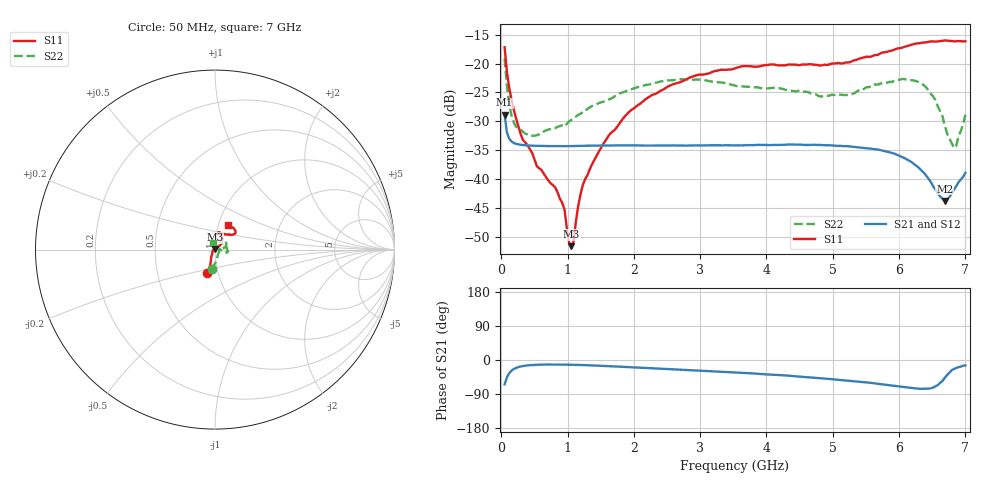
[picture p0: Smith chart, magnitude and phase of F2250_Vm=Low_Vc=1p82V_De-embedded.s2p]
! Integrated Device Technology
! Corporate Headquarters
! 6024 Silver Creek Valley Road
! San Jose, CA 95138  USA
! Phone:  1-408-284-8200
! Toll Free:  1-800-223-1366
! Webpage:  http://www.idt.com/
! Timing and RF Division
! 515 Groton Road, Suite 102
! Westford, MA 01886-6024
! Device:  F2250
! Description: Voltage Variable RF Attenuator
! Frequency:  50.0 -  6000.00 MHz
! Package:  3x3 mm Thin QFN Plastic Package: 16 pin
! Ports:  2 RF, 3 DC
!  Pin  1  = GND
!  Pin  2  = NC
!  Pin  3  = RF1  = Port 1
!  Pin  4  = NC
!  Pin  5  = GND
!  Pin  6  = GND
!  Pin  7  = GND
!  Pin  8  = GND
!  Pin  9  = NC
!  Pin 10  = RF2  = Port 2
!  Pin 11  = NC
!  Pin 12  = GND
!  Pin 13  = GND
!  Pin 14  = VCNTRL
!  Pin 15  = VDD
!  Pin 16  = VMODE
! Vcntrl:  1.820 Volts
! Vmode:  +0.000 Volts
! Vdd:  +3.30  Volts
! Current:  1.186 mA
! Data:  The device was measured on a the F2250 evaluation board which has
!  individual transmission lines to the RF pins.  Data was collected
!  using a calibrated network analyzer.  The evaluation board was
!  de-embedded using a TRL calibration technique.
!  The reference plane is the edge of the package pin.
! Misc:  SN 10
!  Action Tracker AT0258
! Date Measured:  2014-11-26
! Date:  2015-10-15  MJV
! Note:
!  Integrated Device Technology supplies this data as a sample of measured
!  data at the package pin for this product.  Your particular data for this
!  product may vary.
!  Data was taken at 25 degrees C.
!  Integrated Device Technology reserves the right to change this data at anytime.
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# GHz S dB R 50
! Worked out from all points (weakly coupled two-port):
!   201 points, 50 MHz to 7 GHz, reference 50 ohm
!   highest |S21| = -28.84 dB at 50 MHz (marker M1); lowest = -43.8 dB at 6.687 GHz (marker M2)
!   lowest |S11| = -51.6 dB at 1.058 GHz (marker M3), VSWR 1.01, Z = 49.9 + j0.233 ohm
!   |S11| at or under -10 dB: start of sweep to end of sweep
!   |S22| runs from -34.6 to -19.1 dB; largest |S21 - S12| = 5.5e-05
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0.05  -17.17 -108.4  -28.84 -64.2  -28.84 -64.2  -19.11 -100.0
0.1195  -24.20 -111.4  -33.00 -34.7  -33.01 -34.7  -26.93 -73.8
0.22375  -29.54 -121.5  -33.90 -20.8  -33.90 -20.8  -30.94 -50.6
0.5365  -37.77 -154.4  -34.25 -12.6  -34.24 -12.6  -32.40 -9.2
0.91875  -44.10 158.0  -34.30 -12.2  -34.29 -12.2  -30.70 -0.4
0.9535  -45.28 170.4  -34.30 -12.2  -34.29 -12.2  -30.90 1.8
1.023  -51.05 141.9  -34.29 -12.4  -34.29 -12.4  -30.02 4.1
1.05775  -51.61 117.1  -34.28 -12.5  -34.28 -12.5  -29.75 5.0
1.0925  -50.74 83.0  -34.27 -12.7  -34.27 -12.7  -29.50 4.7
1.162  -44.50 53.3  -34.26 -13.0  -34.26 -13.0  -28.88 4.0
1.2315  -40.95 42.1  -34.24 -13.3  -34.25 -13.3  -28.39 4.0
1.6485  -32.07 41.2  -34.19 -16.4  -34.19 -16.4  -26.09 12.4
2.37825  -24.88 47.0  -34.19 -22.6  -34.18 -22.7  -23.19 23.1
3.525  -20.83 72.3  -34.17 -32.9  -34.17 -33.0  -23.84 50.8
4.7065  -20.19 72.2  -34.05 -46.5  -34.06 -46.6  -25.24 56.6
5.22775  -19.81 56.2  -34.31 -54.6  -34.30 -54.6  -25.42 31.9
5.85325  -17.83 40.3  -35.38 -66.6  -35.37 -66.6  -23.19 0.0
6.3745  -16.34 41.3  -38.91 -76.0  -38.92 -76.1  -23.75 -14.3
6.54825  -16.20 45.1  -41.83 -69.6  -41.84 -69.7  -26.35 -15.4
6.68725  -16.00 48.7  -43.78 -47.6  -43.80 -47.1  -30.63 1.7
6.82625  -16.15 53.5  -41.84 -23.9  -41.80 -23.8  -34.59 49.1
7  -16.14 63.2  -38.91 -14.4  -38.88 -14.3  -28.85 103.8
